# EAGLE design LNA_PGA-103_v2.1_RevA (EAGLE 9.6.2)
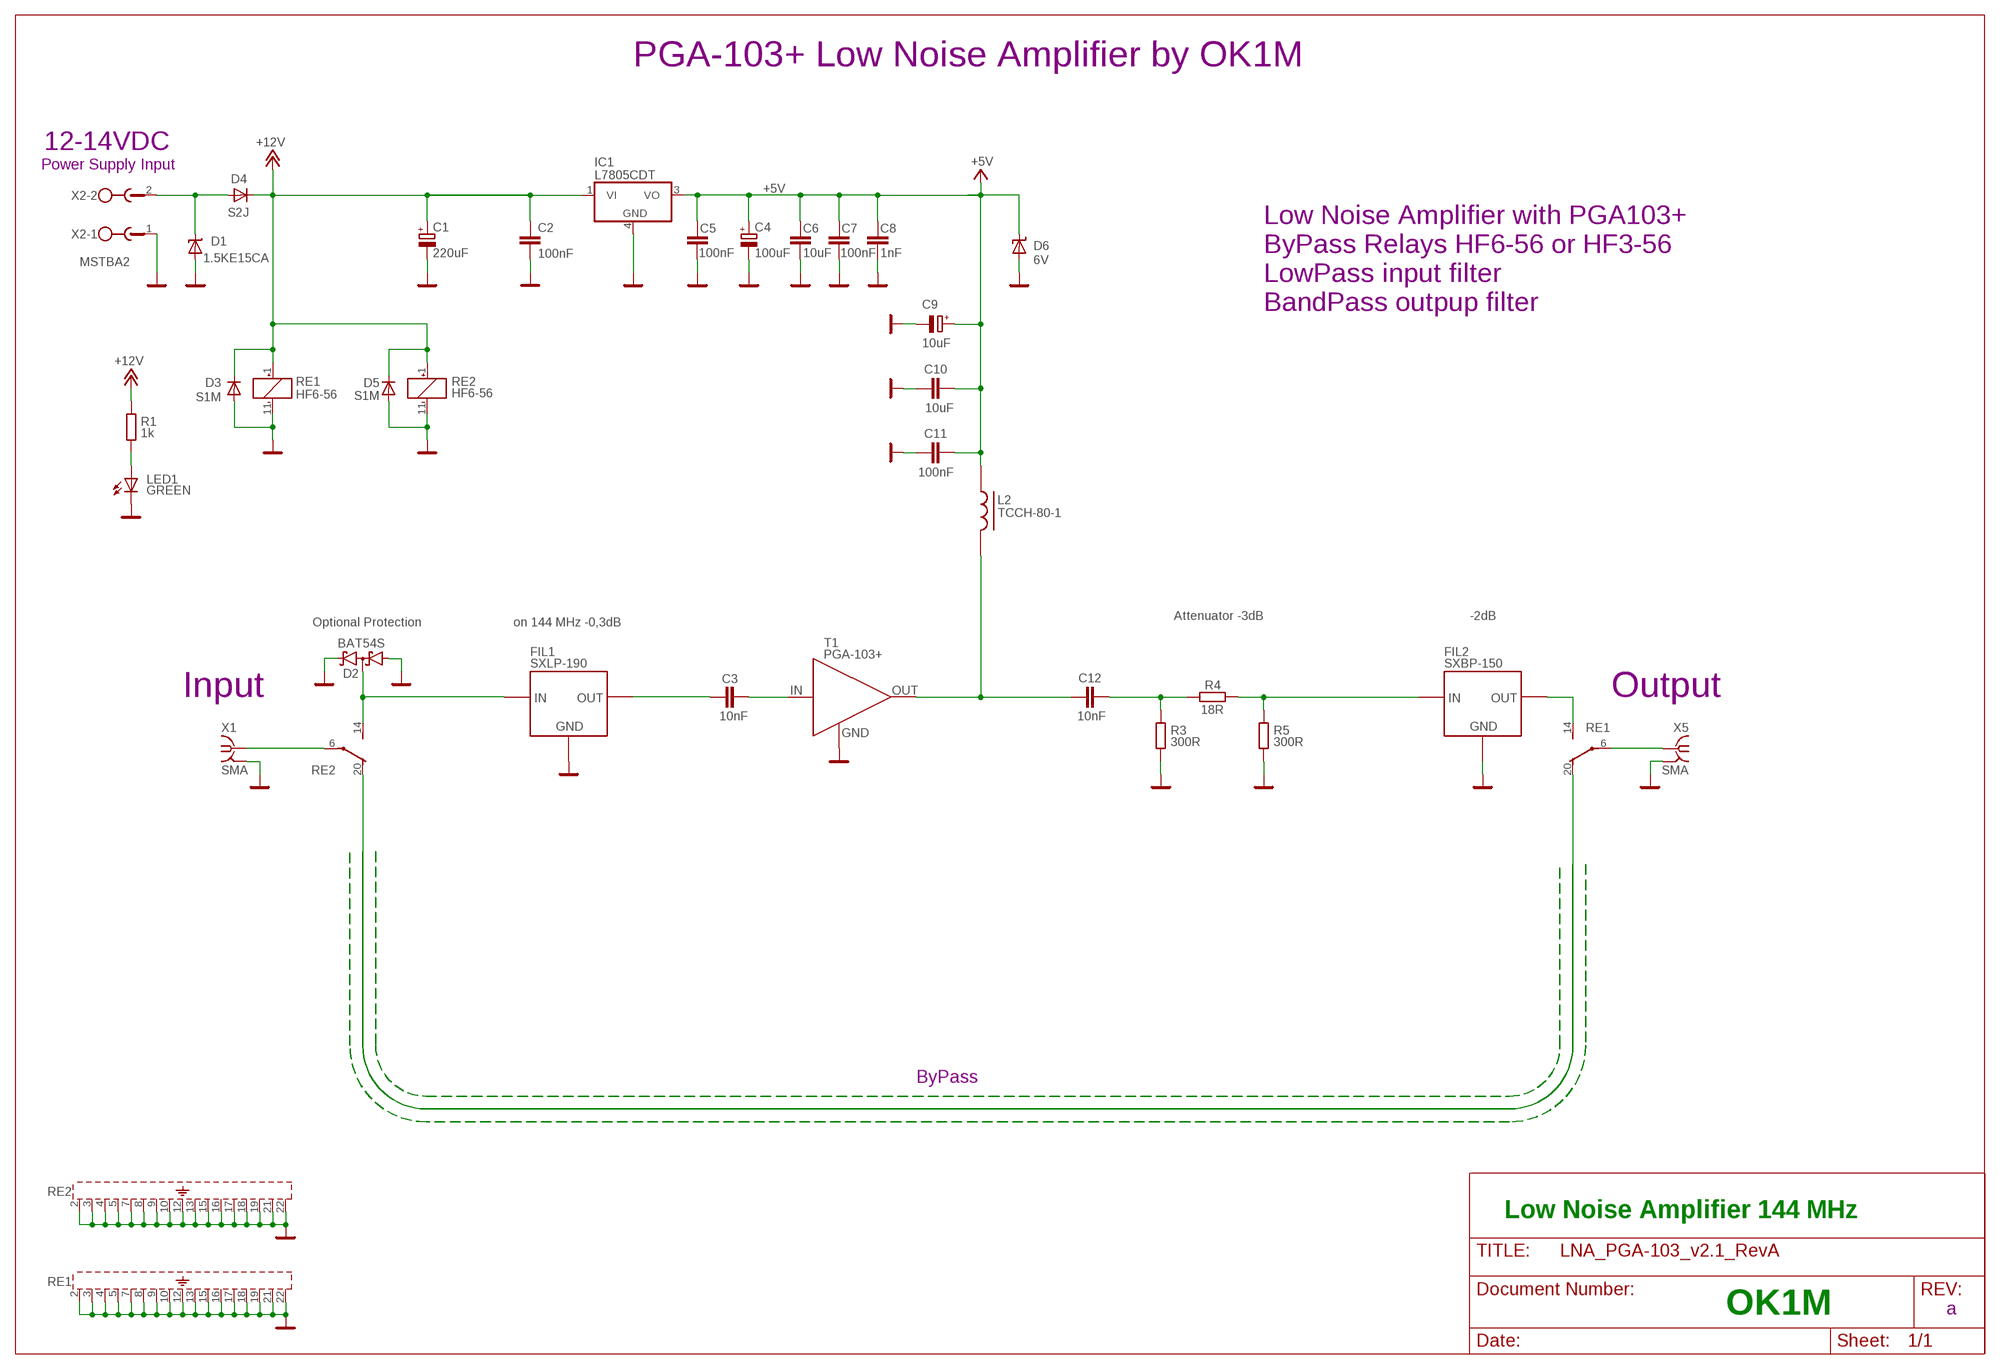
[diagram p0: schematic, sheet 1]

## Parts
C1  220uF  CPOL-EUG  [PANASONIC_G]
C2  100nF  C-EUC0805  [C0805]
C3  10nF  C-EUC0805  [C0805]
C4  100uF  CPOL-EUSMCC  [SMC_C]
C5  100nF  C-EUC0805  [C0805]
C6  10uF  C-EUC0805  [C0805]
C7  100nF  C-EUC0805  [C0805]
C8  1nF  C-EUC0805  [C0805]
C9  10uF  CPOL-EUSMCB  [SMC_B]
C10  10uF  C-EUC1812  [C1812]
C11  100nF  C-EUC0805  [C0805]
C12  10nF  C-EUC0805  [C0805]
D1  1.5KE15CA  TRANSILC2673  [C2673]
D2  BAT54S  [SOT23]
D3  S1M  DIODE-DO-214AC  [DO-214AC]
D4  S2J  DIODE-SMB  [SMB]
D5  S1M  DIODE-DO-214AC  [DO-214AC]
D6  6V  SUPPRESSOR-SMBJ  [SMBJ]
FIL1  SXLP-190  [HF1139]
FIL2  SXBP-150  SXLP-190  [HF1139]
IC1  L7805CDT  MC78M05ABDT  [DPACK_3]
L2  TCCH-80-1  TCCH-80+  [GU1604]
LED1  GREEN  LED3MM  [LED3MM]
R1  1k  R-EU_M0805  [M0805]
R3  300R  R-EU_M1206  [M1206]
R4  18R  R-EU_R1206  [R1206]
R5  300R  R-EU_M1206  [M1206]
RE1  HF6-56  HF6-56+  [HF6-56]
RE2  HF6-56  HF6-56+  [HF6-56]
T1  PGA-103+  [SOT-89]
X1  SMA  SMA-142-0711-881/886  [J502-ND-142-0711-881/886]
X2  MSTBA2  [MSTBA2]
X5  SMA  SMA-142-0711-881/886  [J502-ND-142-0711-881/886]

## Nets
+5V: C4.+ C5.1 C6.1 C7.1 C8.1 C9.+ C10.1 C11.1 D6.C IC1.3(VO) L2.P1
+12V: C1.+ C2.1 D3.C D4.C D5.C IC1.1(VI) R1.2 RE1.1 RE2.1
BYPASS: RE1.20 RE2.20
GND: C1.- C2.2 C4.- C5.2 C6.2 C7.2 C8.2 C9.- C10.2 C11.2 D1.A D2.1(A1) D2.2(C2) D3.A D5.A D6.A FIL1.P$2(GND) FIL1.P$3(GND) FIL1.P$4(GND) FIL1.P$5(GND) FIL1.P$6(GND) FIL1.P$7(GND) FIL2.P$2(GND) FIL2.P$3(GND) FIL2.P$4(GND) FIL2.P$5(GND) FIL2.P$6(GND) FIL2.P$7(GND) IC1.4(GND) LED1.K(C) R3.1 R5.1 RE1.2 RE1.3 RE1.4 RE1.5 RE1.7 RE1.8 RE1.9 RE1.10 RE1.11 RE1.12 RE1.13 RE1.15 RE1.16 RE1.17 RE1.18 RE1.19 RE1.21 RE1.22 RE2.2 RE2.3 RE2.4 RE2.5 RE2.7 RE2.8 RE2.9 RE2.10 RE2.11 RE2.12 RE2.13 RE2.15 RE2.16 RE2.17 RE2.18 RE2.19 RE2.21 RE2.22 T1.2(GND) T1.4(GND) X1.G@1 X1.G@2 X1.G@3 X1.G@4 X2.1 X5.G@1 X5.G@2 X5.G@3 X5.G@4
N$13: D2.3(C1A2) FIL1.INPUT(IN) RE2.14
N$14: FIL2.OUTPUT(OUT) RE1.14
N$15: RE1.6 X5.1
N$16: LED1.A R1.1
N$19: RE2.6 X1.1
N$22: D1.C D4.A X2.2
N$23: C12.2 R3.2 R4.1
N$24: FIL2.INPUT(IN) R4.2 R5.2
T1A: C3.1 FIL1.OUTPUT(OUT)
T1B: C3.2 T1.1(IN)
T1C: C12.1 L2.P3 T1.3(OUT)

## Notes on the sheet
- PGA-103+ Low Noise Amplifier by OK1M
- 12-14VDC
- Power Supply Input
- Low Noise Amplifier with PGA103+
  ByPass Relays HF6-56 or HF3-56
  LowPass input filter
  BandPass outpup filter
- Attenuator -3dB | -2dB
- Optional Protection | on 144 MHz -0,3dB
- Input | Output
- ByPass
- Low Noise Amplifier 144 MHz
- OK1M
- a

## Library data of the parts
C1 C4 C9 = rcl:CPOL-EU: POLARIZED CAPACITOR, European symbol
C2 C3 C5-C8 C10-C12 = rcl:C-EU: CAPACITOR, European symbol
D1 = #Marek:TRANSIL: TRANSIL
D2 = diode:BAT54S: Schottky Diodes Pin connection corrected 2011-05-04 Source: Fairchild .. BAT54.pdf
D3-D5 = diode:DIODE-: DIODE
D6 = diode:SUPPRESSOR-: Suppressor diode
FIL1 FIL2 = #mini-circuit:SXLP-190: PolMar
IC1 = linear:MC78M: 500 mA Positive Voltage Regulators Source: Data sheet
L2 = #mini-circuit:TCCH-80+: PolMar
LED1 = led:LED: LED
R1 R3 R5 = rcl:R-EU_: RESISTOR, European symbol
R4 = rcl:R-EU_: RESISTOR, European symbol; SPICEPREFIX: R
RE1 RE2 = #hf6-56:HF6-56+
T1 = #mini-circuit:PGA-103+: kufmic
X1 X5 = con-coax:SMA-: SMA 50 Ohm End Launch Jack Receptacle - Round Contact; MF: JOHNSON COMPONENTS; MPN: 142-0711-881; OC_FARNELL: unknown; OC_NEWARK: 50B4464
X2 = con-phoenix-508:MSTBA2: PHOENIX; MF: FARNELL; MPN: 1757242; OC_FARNELL: 3705171; OC_NEWARK: 71C4161

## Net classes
0 default: width 0.203 mm, drill 0.406 mm, clearance 0.203 mm

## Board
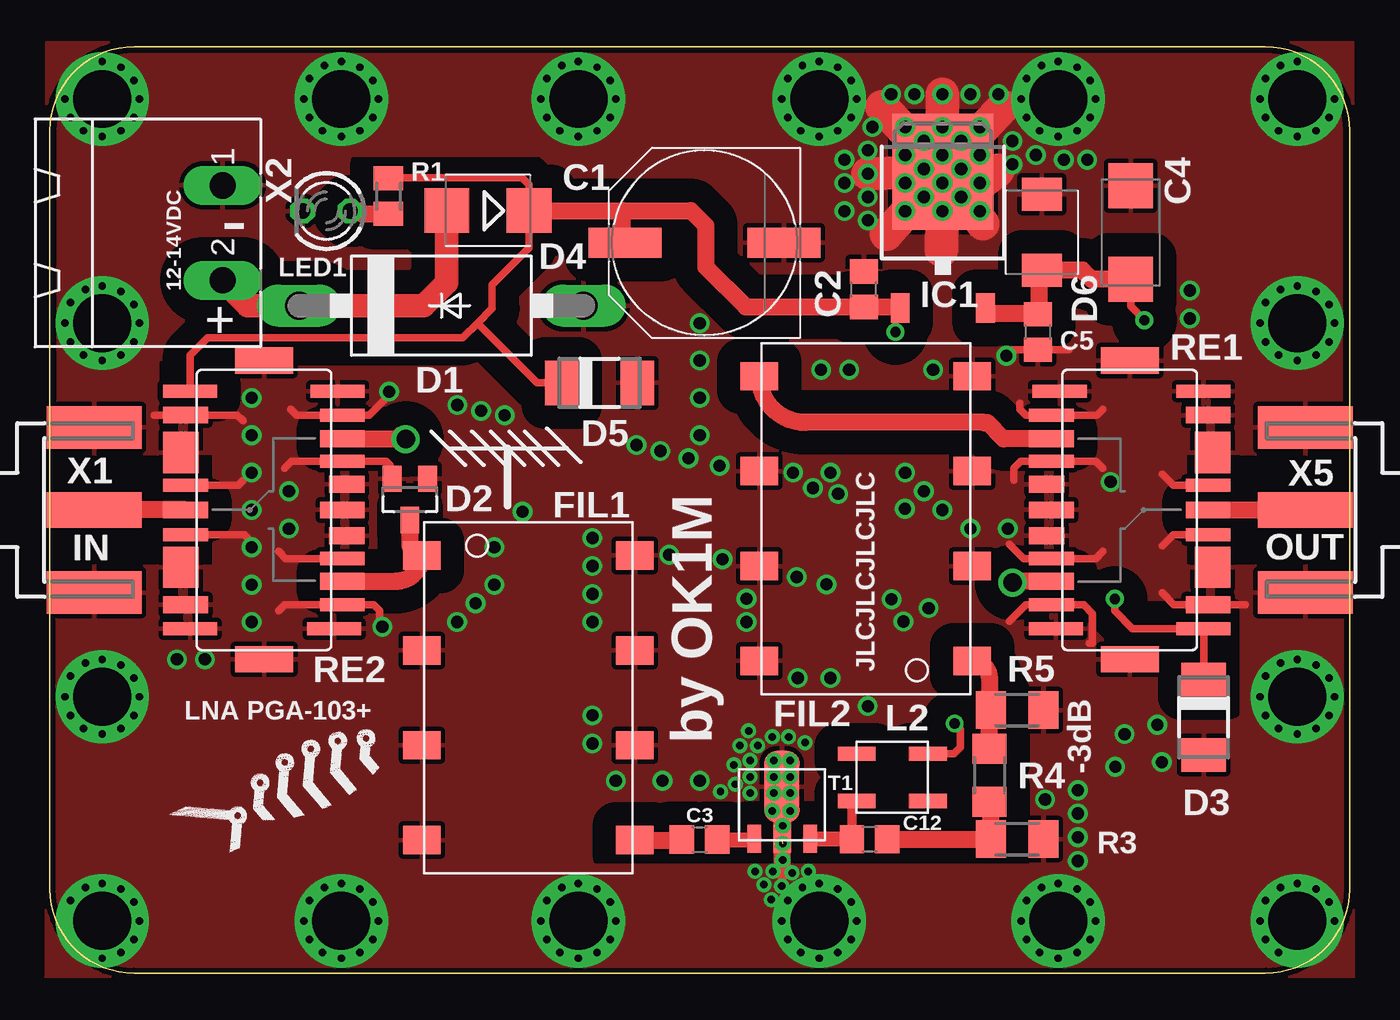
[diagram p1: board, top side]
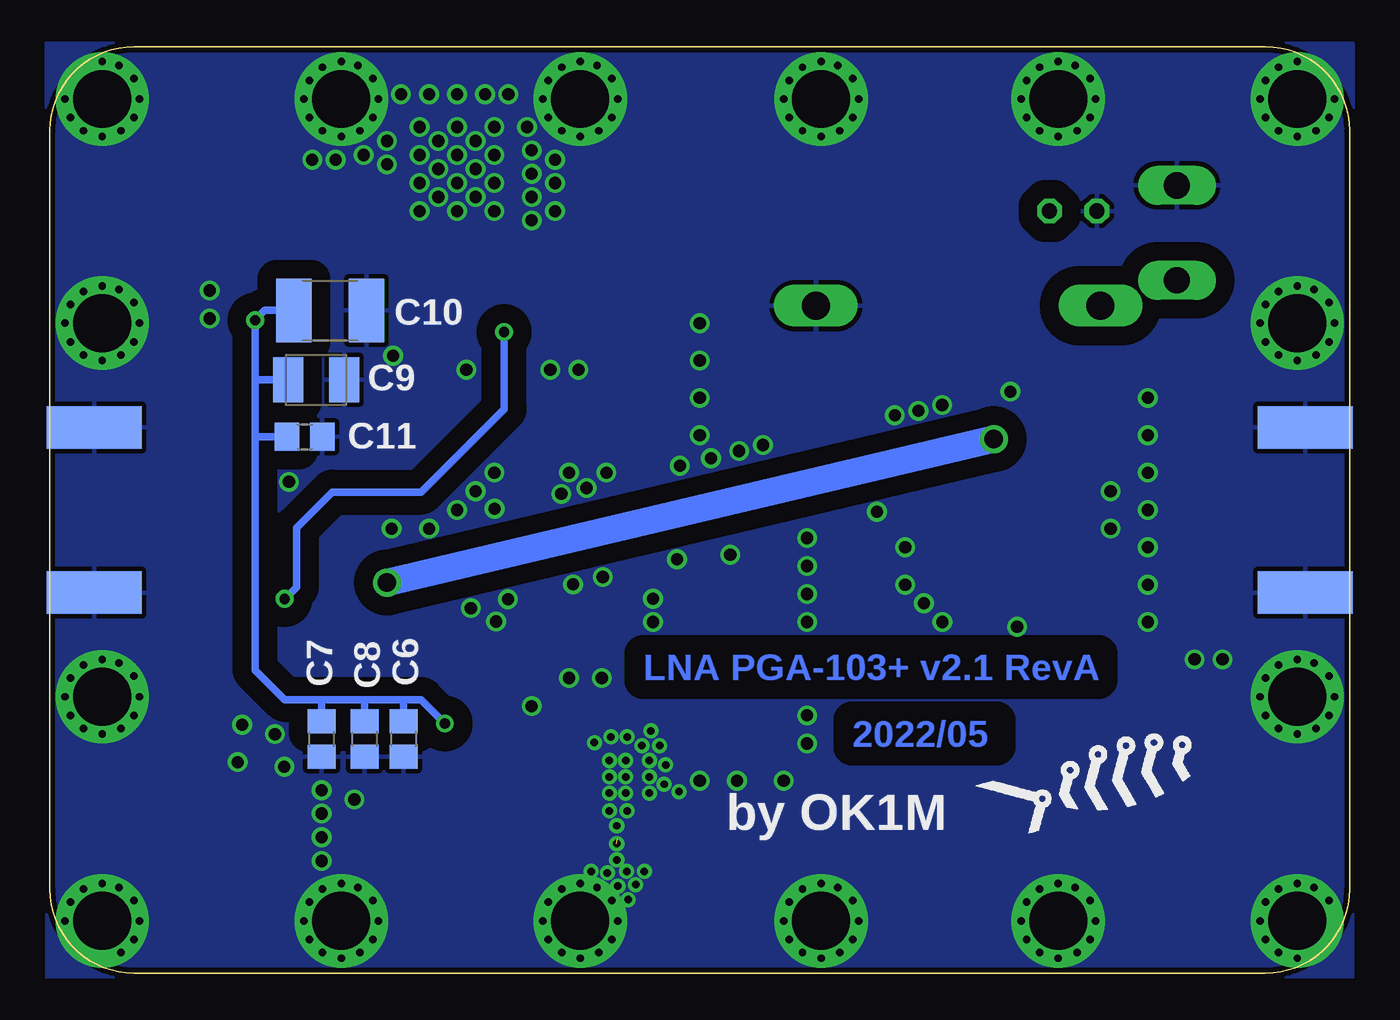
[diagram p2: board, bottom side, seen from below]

Size 69.6 x 49.6 mm. Coordinates in mm from the lower left corner, seen from the top.
Outline: 4.5,0 65.1,0 arc90 69.6,4.5 69.6,45.1 arc90 65.1,49.6 4.5,49.6 arc90 0,45.1 0,4.5 arc90 4.5,0
Copper layers (1*16): Top 0.035mm / dielectric 1.6mm / Bottom 0.035mm
Design rules "JLCPCB_2layer_cheap": minimum track width 5mil, minimum drill 0.2mm, track to track 5mil, track to pad 8mil, pad to pad 8mil, via to via 8mil, smd to smd 8mil, copper to edge 10mil, drill to drill 8mil, minimum pad ring 10mil, minimum via ring 8mil, stop-mask expansion 4mil, vias tented up to drill 0.7mm, thermal gap 10mil

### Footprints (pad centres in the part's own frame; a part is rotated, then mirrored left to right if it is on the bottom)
PANASONIC_G = smd 3.9 x 1.6: + 4.25,0; - -4.25,0
C0805 = smd 1.3 x 1.5: 1 -0.95,0; 2 0.95,0
SMC_C = smd 2.4 x 2.4: + -2.5,0; - 2.5,0
SMC_B = smd 1.6 x 2.4: + -1.5,0; - 1.5,0
C1812 = smd 1.9 x 3.4: 1 -1.95,0; 2 1.95,0
C2673 = drill 1.499 long: A 7.62,0; C -7.62,0
SOT23 = smd 1 x 1.4: 1 -0.95,-1.1; 2 0.95,-1.1; 3 0,1.1
DO-214AC = smd 1.8 x 2.4: A 2.025,0; C -2.025,0
SMB = smd 2.4 x 2.4: A 2.2,0; C -2.2,0
SMBJ = smd 1.78 x 2.16: A 2.04,0; C -2.03,0
HF1139 = smd 1.52 x 2: INPUT -7.62,-5.7; OUTPUT 7.62,5.7; P$2 -7.62,5.7; P$3 -2.54,-5.7; P$4 -2.54,5.7; P$5 2.54,-5.7; P$6 2.54,5.7; P$7 7.62,-5.7
DPACK_3 = smd 1 x 1.6: 1 -2.28,-4.8; 3 2.28,-4.8 | smd 5.4 x 6.2: 4 0,2.5
GU1604 = smd 0.762 x 2.032: P1 -1.27,1.905; P2 1.27,1.905; P3 1.27,-1.905; P4 -1.27,-1.905
LED3MM = drill 0.813 octagon: A -1.27,0; K 1.27,0
M0805 = smd 1.3 x 1.6: 1 -0.95,0; 2 0.95,0
M1206 = smd 1.6 x 2: 1 -1.4,0; 2 1.4,0
R1206 = smd 1.6 x 1.803: 1 -1.422,0; 2 1.422,0
HF6-56 = smd 0.7 x 2.9: 1 -6.35,-3.95; 11 6.35,-3.95; 12 6.35,3.75; 22 -6.35,3.95 | smd 0.9 x 2.4: 2 -5.08,-4.2; 6 0,-4.2; 10 5.08,-4.2; 14 3.81,4.2; 17 0,4.2; 20 -3.81,4.2 | smd 2.2 x 1.9: 3 -3.075,-4.45; 8 3.075,-4.45 | smd 1.4 x 3.1: 4 -8,0; 9 8,0 | smd 0.7 x 2.4: 5 -1.317,-4.2; 7 1.317,-4.2; 13 5.08,4.2; 15 2.6,4.2; 19 -2.6,4.2; 21 -5.08,4.2 | smd 0.9 x 1.9: 16 1.375,4.45; 18 -1.375,4.45
SOT-89 = smd 0.711 x 1.499: 1 -0.457,-1.194; 3 2.54,-1.194 | smd 0.914 x 1.499: 2 1.041,-1.194 | smd 1.905 x 3.81: 4 1.022,1.597
J502-ND-142-0711-881/886 = smd 5.08 x 1.905: 1 2.565,0 | smd 5.08 x 2.286: G@1 2.565,4.42; G@2 2.565,-4.42 | smd 5.08 x 2.286 bottom: G@3 2.565,4.42; G@4 2.565,-4.42
MSTBA2 = drill 1.397 long: 1 -2.54,5.08; 2 2.54,5.08

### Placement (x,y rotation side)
C1  35.05,39.1 180 top
C2  43.58,36.62 90 top
C3  34.78,7.16 0 top
C4  57.87,39.65 90 top
C5  52.9,34.33 270 top
C6  50.66,12.54 270 bottom
C7  55.06,12.54 270 bottom
C8  52.76,12.54 270 bottom
C9  55.34,31.76 0 bottom
C10  54.6,35.48 0 bottom
C11  55.96,28.72 0 bottom
C12  43.89,7.18 0 top
D1  20.96,35.74 0 top
D2  19.27,25.36 180 top
D3  61.78,13.7 270 top
D4  23.45,40.83 180 top
D5  29.43,31.6 0 top
D6  53.12,39.66 90 top
FIL1  25.62,14.75 270 top
FIL2  43.69,24.34 90 top
IC1  47.82,40.41 0 top
L2  45.11,10.48 270 top
LED1  14.8,40.8 180 top
R1  18.13,41.6 90 top
R3  51.8,7.18 180 top
R4  50.31,10.6 90 top
R5  51.8,14.09 180 top
RE1  57.82,24.8 90 top
RE2  11.46,24.8 270 top
T1  38.17,8.39 0 top
U$1  [RYBICKA_12MM]  13.7,10.03 10 top
U$2  [RYBICKA_12MM]  12.58,10.28 0 bottom
X1  -0.2,24.8 0 top
X2  4.16,39.63 270 top
X5  69.8,24.8 180 top

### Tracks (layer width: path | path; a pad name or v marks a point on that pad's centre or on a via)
+5V  (via drill 0.55)
  Top 0.203: C5.1 52.9,37.41 D6.C
  Top 0.406: L2.P1 48.42,11.75 48.77,12.1 48.77,13.05 v48.45,13.37 | v58.61,34.96 57.87,35.7 C4.+
  Top 0.9: IC1.3 50.42,35.29 52.91,35.29 52.97,35.35 52.97,37.48 D6.C 55.3,37.63 55.79,37.15 C4.+
  Bottom 0.406: v48.45,13.37 49.72,14.64 50.67,14.64 | 50.67,14.64 52.9,14.64 | 52.9,14.64 55.12,14.64 | 55.12,14.64 57.02,14.64 58.61,16.23 58.61,28.61 | 58.61,28.61 58.61,31.79 | 58.61,31.79 v58.61,34.96 58.09,35.48 C10.1 | C6.1 50.66,14.62 50.67,14.64 | C8.1 52.76,14.5 52.9,14.64 | C7.1 55.06,14.58 55.12,14.64 | C11.1 58.51,28.72 58.61,28.61 | C9.+ 58.59,31.76 58.61,31.79
+12V  (via drill 0.55)
  Top 0.406: R1.2 18.15,42.58 25.27,42.58 25.65,42.2 D4.C 25.65,38.83 23.69,36.87 23.69,35.59 22.89,34.8 | RE2.1 7.51,33.08 8.45,34.01 22.1,34.01 22.89,34.8 | D5.C 26.1,31.6 22.89,34.8 | D3.C 61.78,18.44 RE1.1 57.98,18.45 57.02,19.4 v57.02,20.04 | v45.28,34.33 45.28,35.35 IC1.1
  Top 0.9: D4.C 30.67,40.83 | 30.67,40.83 34.33,40.83 35.12,40.04 35.12,37.82 37.27,35.67 C2.1 45.48,35.67 IC1.1 | C1.+ 30.67,39.23 30.67,40.83
  Bottom 0.406: v57.02,20.04 56.39,20.67 56.39,23.85 54.48,25.75 49.72,25.75 45.28,30.2 v45.28,34.33
BYPASS  (via drill 1)
  Top 0.9: RE1.20 51.55,20.99 v51.55,20.91 | RE2.20 18.8,28.61 18.8,28.8 19.06,28.8
  Top 1: 19.06,28.8 v19.06,28.59
  Bottom 0.9: 51.71,20.83 51.63,20.83 v51.55,20.91
  Bottom 1.5: v19.06,28.59 v51.55,20.91
GND  (via drill 0.4, 0.65, 3.1 pad 5)  (1 unrouted)
  Top 0.406: RE2.5 10.08,26.12 10.35,26.39 | 10.35,29.56 10.03,29.88 RE2.2 5.59,29.88 | RE2.7 10.4,23.48 10.67,23.21 | RE2.15 12.63,22.2 12.26,22.58 | 12.26,19.4 12.57,19.72 RE2.13 17.34,19.72 17.65,19.4 17.65,18.77 | 12.57,27.02 12.95,27.4 RE2.19 17.99,27.4 18.21,27.18 | 12.89,30.2 13.21,29.88 RE2.21 17.1,29.88 17.89,30.67 | 51.94,30.52 51.94,30.2 52.26,29.88 RE1.13 56.07,29.88 56.39,30.2 | 56.39,27.02 56.01,27.4 RE1.15 52,27.4 51.63,27.02 51.63,26.39 | 51.39,22.97 52.16,22.2 RE1.19 56.01,22.2 56.39,22.58 | 51.39,18.85 52.26,19.72 RE1.21 55.36,19.72 55.83,19.24 55.83,17.66 55.68,17.66 | 59.56,20.36 60.2,19.72 RE1.2 64.01,19.72 | RE1.5 60.15,23.48 59.56,22.89 | RE1.7 60.15,26.12 59.56,26.71 | v51.22,33.05 51.54,33.37 54.56,33.37
  Top 0.9: T1.4 39.2,5.48 39.24,5.43
  Top 1.8: v47.8,47.05 47.81,44.8 IC1.4 | IC1.4 v43.8,42.8 | IC1.4 50.75,42.98 v47.8,40.8 | IC1.4 47.74,38.69 v47.8,42.3 | IC1.4 44.56,46.39 | IC1.4 51.07,46.39 | IC1.4 49.96,40.12 | IC1.4 44.8,39.56
  other vias: 2.8,34.8 0.8,34.8 4.8,34.8 2.8,36.8 2.8,32.8 1.1,33.8 1.8,33.1 3.8,33.1 4.5,33.8 4.5,35.8 3.8,36.5 1.9,36.6 1.1,35.9 2.8,46.8 0.8,46.8 4.8,46.8 2.8,48.8 2.8,44.8 1.1,45.8 1.8,45.1 3.8,45.1 4.5,45.8 4.5,47.8 3.8,48.5 66.8,46.8 64.8,46.8 68.8,46.8 66.8,48.8 66.8,44.8 65.1,45.8 65.8,45.1 67.8,45.1 68.5,45.8 65.9,48.6 65.1,47.9 66.8,34.8 64.8,34.8 68.8,34.8 66.8,36.8 66.8,32.8 65.1,33.8 65.8,33.1 67.8,33.1 68.5,33.8 68.5,35.8 67.8,36.5 65.9,36.6 65.1,35.9 66.8,14.8 64.8,14.8 68.8,14.8 66.8,16.8 66.8,12.8 65.1,13.8 65.8,13.1 67.8,13.1 68.5,13.8 68.5,15.8 67.8,16.5 65.9,16.6 65.1,15.9 66.8,2.8 64.8,2.8 68.8,2.8 66.8,4.8 65.1,1.8 65.8,1.1 68.5,3.8 67.8,4.5 65.9,4.6 65.1,3.9 2.8,2.8 4.8,2.8 2.8,4.8 2.8,0.8 3.8,1.1 4.5,1.8 4.5,3.8 3.8,4.5 1.9,4.6 1.1,3.9 15.6,2.8 13.6,2.8 17.6,2.8 15.6,4.8 15.6,0.8 13.9,1.8 14.6,1.1 16.6,1.1 17.3,1.8 17.3,3.8 16.6,4.5 14.7,4.6 13.9,3.9 28.3,2.8 26.3,2.8 30.3,2.8 28.3,4.8 28.3,0.8 26.6,1.8 27.3,1.1 29.3,1.1 30,1.8 30,3.8 29.3,4.5 27.4,4.6 26.6,3.9 41.2,2.8 39.2,2.8 43.2,2.8 41.2,4.8 41.2,0.8 39.5,1.8 40.2,1.1 42.2,1.1 42.9,1.8 42.9,3.8 42.2,4.5 40.3,4.6 39.5,3.9 54,2.8 52,2.8 56,2.8 54,4.8 54,0.8 52.3,1.8 53,1.1 55,1.1 55.7,1.8 55.7,3.8 55,4.5 53.1,4.6 52.3,3.9 15.6,46.8 13.6,46.8 17.6,46.8 15.6,48.8 15.6,44.8 13.9,45.8 14.6,45.1 16.6,45.1 17.3,45.8 17.3,47.8 16.6,48.5 14.7,48.6 13.9,47.9 28.3,46.8 26.3,46.8 30.3,46.8 28.3,48.8 28.3,44.8 26.6,45.8 27.3,45.1 29.3,45.1 30,45.8 30,47.8 29.3,48.5 27.4,48.6 26.6,47.9 41.2,46.8 39.2,46.8 43.2,46.8 41.2,48.8 41.2,44.8 39.5,45.8 40.2,45.1 42.2,45.1 42.9,45.8 42.9,47.8 42.2,48.5 40.3,48.6 39.5,47.9 54,46.8 52,46.8 56,46.8 54,48.8 54,44.8 52.3,45.8 53,45.1 55,45.1 55.7,45.8 55.7,47.8 55,48.5 53.1,48.6 52.3,47.9 2.8,14.8 0.8,14.8 4.8,14.8 2.8,16.8 2.8,12.8 1.1,13.8 1.8,13.1 3.8,13.1 4.5,13.8 4.5,15.8 3.8,16.5 1.9,16.6 1.1,15.9 37.42,12.97 36.94,12.18 37.9,12.18 37.5,11.39 36.63,11.15 37.5,10.51 36.7,10.12 37.5,9.64 35.91,9.72 38.77,11.39 38.77,10.51 38.77,9.64 38.69,8.69 39.24,7.89 39.24,6.94 39.24,6.07 39.64,8.69 39.64,9.64 39.64,10.51 39.64,11.39 38.69,12.66 39.56,12.66 40.44,12.34 10.8,24.8 10.8,22.8 10.8,20.8 10.8,18.8 10.8,26.8 10.8,28.8 10.8,30.8 12.8,25.8 12.8,23.8 23.8,22.8 23.8,20.8 21.8,18.8 34.8,34.8 34.8,32.8 34.8,30.8 34.8,28.8 39.8,26.8 45.8,26.8 41.8,26.8 41.3,32.3 42.8,32.3 47.3,32.3 46.8,25.8 47.8,24.8 51.3,23.8 49.3,23.8 43.8,14.3 34.8,10.3 32.8,10.3 30.3,10.3 8.3,16.8 6.8,16.8 22.8,19.8 17.8,18.55 29.05,23.3 29.05,21.8 29.05,20.3 29.05,18.8 29.05,13.8 29.05,12.3 37.3,20.05 37.3,18.8 40.05,15.8 41.8,15.8 53.3,9.3 55.05,9.8 57.55,12.8 57.05,11.05 59.3,13.3 59.55,11.3 55.05,8.55 56.8,26.3 61.05,35.05 61.05,36.55 45.8,45.3 47.8,45.3 49.8,45.3 45.8,43.8 47.8,43.8 49.8,43.8 48.8,44.55 46.8,44.55 45.05,47.05 46.3,47.05 49.3,47.05 50.8,47.05 51.55,44.55 44.05,45.3 43.8,44.05 43.8,41.55 43.8,40.3 42.55,42.3 42.55,43.55 42.55,40.8 51.55,43.3 46.8,43.05 48.8,43.05 49.8,42.3 45.8,42.3 46.8,41.55 48.8,41.55 49.8,40.8 45.8,40.8 52.8,43.8 54.3,43.55 55.55,43.55 38.71,5.45 39.75,5.37 37.76,5.45 38.24,4.74 39.19,4.66 40.62,5.45 38.63,3.94 55.05,7.28 55.05,6.01 21.82,30.42 23.09,30.1 24.36,29.86 31.42,28.28 32.69,27.96 34.2,27.56 35.86,27.17 25.31,24.71 39.99,21.21 41.58,20.82 45.07,20.02 47.06,19.55 45.79,24.86 42.21,25.66 40.87,25.98 45.71,18.83 36.02,22.16 33.17,22.4 18.16,31.13
  pour Top: -0.2,-0.2 -0.2,21.8 5.8,21.8 5.8,5.8 63.8,5.8 63.8,21.8 69.8,21.8 69.8,-0.2
  pour Top (isolate 0.305): -0.2,27.8 5.8,27.8 5.8,43.8 63.8,43.8 63.8,27.8 69.8,27.8 69.8,49.8 -0.2,49.8
  pour Bottom: -0.2,24.8 5.8,24.8 5.8,39.3 arc-90 10.3,43.8 63.8,43.8 63.8,24.8 69.8,24.8 69.8,49.8 -0.2,49.8
  pour Bottom: -0.2,24.8 5.8,24.8 5.8,5.8 63.8,5.8 63.8,24.8 69.8,24.8 69.8,-0.2 -0.2,-0.2
  pour Bottom (isolate 1): 4.8,4.8 4.8,21.8 5.8,21.8 5.8,27.8 4.8,27.8 4.8,44.8 63.8,44.8 63.8,4.8
  pour Top (isolate 1.27): 4.8,4.8 4.8,21.8 8.8,21.8 8.8,27.8 4.8,27.8 4.8,44.8 64.8,44.8 64.8,27.8 60.8,27.8 60.8,21.8 64.8,21.8 64.8,4.8
N$13
  Top 0.9: RE2.14 18.54,20.99 arc90 FIL1.INPUT arc-90 19.27,23.01 D2.3
N$14
  Top 0.9: RE1.14 51.07,28.61 50.2,29.48 arc-90 50.04,29.48 40.47,29.48 arc-90 FIL2.OUTPUT
N$15
  Top 0.9: RE1.6 X5.1
N$16
  Top 0.9: LED1.A 16.58,40.8 16.72,40.65 R1.1
N$19
  Top 0.9: RE2.6 X1.1
N$22
  Top 1.27: X2.2 10.6,35.74 D1.C 20.02,35.74 21.25,36.97 D4.A
N$23
  Top 0.9: C12.2 R3.2 50.4,9.09 arc90 R4.1
N$24
  Top 0.9: R4.2 50.31,14 | 50.31,14 arc-90 R5.2 | FIL2.INPUT arc-90 50.31,15.8 50.31,14
T1A
  Top 0.9: FIL1.OUTPUT 33.8,7.13 arc90 C3.1
T1B
  Top 0.813: C3.2 37.6,7.16 37.64,7.2 arc90 T1.1
T1C
  Top 0.508: C12.1 42.94,8.95 arc-90 L2.P3
  Top 0.813: T1.3 42.93,7.2 arc-90 C12.1

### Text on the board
Bottom: LNA PGA-103+ v2.1 RevA | 2022/05
tPlace: - | + | IN | OUT | JLCJLCJLCJLC | LNA PGA-103+ | -3dB
bPlace: by OK1M
tNames: 12-14VDC | by OK1M
tStop: 2022/05 | 5V | RevA | aCeluto!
